(* Logix 5000 AddOnInstructionDefinition export Banner_K50_Select_Touch_PD_v4; software revision 33.03 *)

TYPE Banner_K50Select_Touch_4State_v4 :   // Process Data for Four State Mode.
STRUCT
   PDI_Output_Status : SINT;   // 0 = Inactive, 1 = Active. Related parameters defined in output and touch setting parameter data.
   PDI_State : SINT;   // 0 = State 1, 1 = State 2, 2 = State 3, 3 = State 4. Animation State. Related parameters defined in four state full logic/mulicolor parameter data.
   PDO_Job_Control : SINT;   // 0 = Off, 1 = On. Job input for 4 state full logic mode.
END_STRUCT
END_TYPE

TYPE Banner_K50Select_Touch_Adv_v4 :   // Advanced Process Data information.
STRUCT
   PDI_Output_Status : SINT;   // 0 = Inactive, 1 = Active. Related parameters defined in output and touch settings parameter data.
   Animation_Type : SINT;   // 0 = Off, 1 = Steady, 2 = Flash, 3 = Two Color Flash, 4 = 50/50, 5 = 50/50 Rotate, 6 = Chase, 7 = Intensity Sweep, 8 = Color Sweep, 9 = Sequence, 10 = Wave, 11 = Double Wave.
   Direction : SINT;   // 0 = CCW, 1 = CW.
   Pattern : SINT;   // 0 = Flash, 1 = Strobe, 2 = Three Pulse, 3 = SOS, 4 = Random.
   Speed : SINT;   // 0 = Slow, 1 = Medium, 2 = Fast, 3 = Custom.
   Static_Sequence : INT;   // 0 to 255. Value describing the LED position on the device.
   Sequence_Start_Location : SINT;   // 0 = LED 1, 1 = LED 2, 2 = LED 3, 3 = LED 4, 4 = LED 5, 5 = LED 6, 6 = LED 7, 7 = LED 8.
   Color_1 : SINT;   // 0 = Green, 1 = Red, 2 = Orange, 3 = Amber, 4 = Yellow, 5 = Lime Green, 6 = Spring Green, 7 = Cyan, 8 = Sky Blue, 9 = Blue, 10 = Violet, 11 = Magenta, 12 = Rose, 13 = White, 14 = Custom 1, 15 = Custom 2.
   Color_1_Intensity : SINT;   // 0 = High, 1 = Medium, 2 = Low, 3 = Off, 4 = Custom.
   Color_2 : SINT;   // 0 = Green, 1 = Red, 2 = Orange, 3 = Amber, 4 = Yellow, 5 = Lime Green, 6 = Spring Green, 7 = Cyan, 8 = Sky Blue, 9 = Blue, 10 = Violet, 11 = Magenta, 12 = Rose, 13 = White, 14 = Custom 1, 15 = Custom 2.
   Color_2_Intensity : SINT;   // 0 = High, 1 = Medium, 2 = Low, 3 = Off, 4 = Custom.
END_STRUCT
END_TYPE

TYPE Banner_K50Select_Touch_LEDControl_v4 :   // LED Control Process Data for a K50 Select.
STRUCT
   PDI_Output_Status : SINT;   // 0 = Inactive, 1 = Active. Related parameters defined in output and touch settings parameter data.
   LED_1_Color : SINT;   // 0 = Green, 1 = Red, 2 = Orange, 3 = Amber, 4 = Yellow, 5 = Lime Green, 6 = Spring Green, 7 = Cyan, 8 = Sky Blue, 9 = Blue, 10 = Violet, 11 = Magenta, 12 = Rose, 13 = White, 14 = Custom 1, 15 = Custom 2.
   LED_1_Intensity : SINT;   // 0 to 10 (0 to 100%).
   LED_2_Color : SINT;   // 0 = Green, 1 = Red, 2 = Orange, 3 = Amber, 4 = Yellow, 5 = Lime Green, 6 = Spring Green, 7 = Cyan, 8 = Sky Blue, 9 = Blue, 10 = Violet, 11 = Magenta, 12 = Rose, 13 = White, 14 = Custom 1, 15 = Custom 2.
   LED_2_Intensity : SINT;   // 0 to 10 (0 to 100%).
   LED_3_Color : SINT;   // 0 = Green, 1 = Red, 2 = Orange, 3 = Amber, 4 = Yellow, 5 = Lime Green, 6 = Spring Green, 7 = Cyan, 8 = Sky Blue, 9 = Blue, 10 = Violet, 11 = Magenta, 12 = Rose, 13 = White, 14 = Custom 1, 15 = Custom 2.
   LED_3_Intensity : SINT;   // 0 to 10 (0 to 100%).
   LED_4_Color : SINT;   // 0 = Green, 1 = Red, 2 = Orange, 3 = Amber, 4 = Yellow, 5 = Lime Green, 6 = Spring Green, 7 = Cyan, 8 = Sky Blue, 9 = Blue, 10 = Violet, 11 = Magenta, 12 = Rose, 13 = White, 14 = Custom 1, 15 = Custom 2.
   LED_4_Intensity : SINT;   // 0 to 10 (0 to 100%).
   LED_5_Color : SINT;   // 0 = Green, 1 = Red, 2 = Orange, 3 = Amber, 4 = Yellow, 5 = Lime Green, 6 = Spring Green, 7 = Cyan, 8 = Sky Blue, 9 = Blue, 10 = Violet, 11 = Magenta, 12 = Rose, 13 = White, 14 = Custom 1, 15 = Custom 2.
   LED_5_Intensity : SINT;   // 0 to 10 (0 to 100%).
   LED_6_Color : SINT;   // 0 = Green, 1 = Red, 2 = Orange, 3 = Amber, 4 = Yellow, 5 = Lime Green, 6 = Spring Green, 7 = Cyan, 8 = Sky Blue, 9 = Blue, 10 = Violet, 11 = Magenta, 12 = Rose, 13 = White, 14 = Custom 1, 15 = Custom 2.
   LED_6_Intensity : SINT;   // 0 to 10 (0 to 100%).
   LED_7_Color : SINT;   // 0 = Green, 1 = Red, 2 = Orange, 3 = Amber, 4 = Yellow, 5 = Lime Green, 6 = Spring Green, 7 = Cyan, 8 = Sky Blue, 9 = Blue, 10 = Violet, 11 = Magenta, 12 = Rose, 13 = White, 14 = Custom 1, 15 = Custom 2.
   LED_7_Intensity : SINT;   // 0 to 10 (0 to 100%).
   LED_8_Color : SINT;   // 0 = Green, 1 = Red, 2 = Orange, 3 = Amber, 4 = Yellow, 5 = Lime Green, 6 = Spring Green, 7 = Cyan, 8 = Sky Blue, 9 = Blue, 10 = Violet, 11 = Magenta, 12 = Rose, 13 = White, 14 = Custom 1, 15 = Custom 2.
   LED_8_Intensity : SINT;   // 0 to 10 (0 to 100%).
   Vibration_Feedback : SINT;   // 0 = Off, 1 = On, 2 = Pattern.
   Vibration_Pattern : SINT;   // 0 = Off, 1 = On, 2 = 3 Pulses, 3 = SOS, 4 = Random.
   Vibration_Speed : SINT;   // 0 = Slow, 1 = Medium, 2 = Fast, 3 = Custom.
END_STRUCT
END_TYPE

TYPE Banner_K50Select_Touch_MC_v4 :   // Process Data for Multicolor
STRUCT
   PDI_Output_State : SINT;   // 0 = Inactive, 1 = Active. Related parameters defined in output and touch setting parameter data.
   PDI_State : SINT;   // 0 = State 1, 1 = State 2, 2 = State 3, 3 = State 4. Animation State. Related parameters defined in four state full logic/mulicolor parameter data.
   PDO_State : SINT;   // 0 = State 1, 1 = State 2, 2 = State 3, 3 = State 4. Animation State. Related parameters defined in four state full logic/mulicolor parameter data.
END_STRUCT
END_TYPE

TYPE Banner_K50Select_Touch_PDIO_v4 :   // UDT that records the converted prcoess data.
STRUCT
   PD_MultiColor : Banner_K50Select_Touch_MC_v4;   // Only active when Operation Mode set to 0. State tells the light which of the four states it should be in. 0 = State 1, 1 = State 2, 2 = State 3, 3 = State 4.
   PD_4State : Banner_K50Select_Touch_4State_v4;   // Only active when Operation Mode set to 1. Job Input tells the light how it should behave. 0 - Off, 1 = ON
   PD_Advanced : Banner_K50Select_Touch_Adv_v4;   // Only active when Operation Mode set to 2.
   PD_LED : Banner_K50Select_Touch_LEDControl_v4;   // Only active when Operation Mode set to 3.
   PDO_DT : SINT[8];
   PDI_DT : SINT[2];
END_STRUCT
END_TYPE

ADD_ON_INSTRUCTION Banner_K50_Select_Touch_PD_v4   (* revision 4.0, vendor Banner Engineering *)
// Takes the raw SINT information and converts that data into actual information.
VAR_IN_OUT
   PD : Banner_K50Select_Touch_PDIO_v4; {required}
END_VAR
VAR_INPUT
   Operation_Mode : SINT; {required}   // Linked from Parameters AOI or entered manually.
   Byte_Swap : BOOL; {required}
END_VAR
VAR
   PDO_Temp : SINT[8]; {access None}
   PDI_Temp : SINT[2]; {access None}
END_VAR

ROUTINE Logic   (* ladder *)
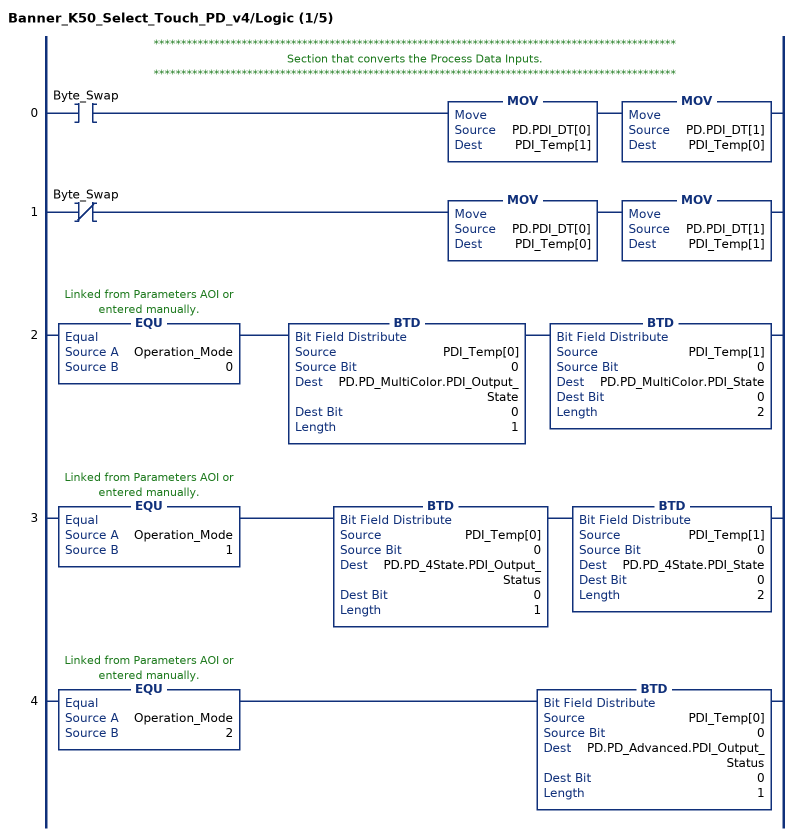
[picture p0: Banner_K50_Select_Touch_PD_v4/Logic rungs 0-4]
   // ***********************************************************************************************
   // Section that converts the Process Data Inputs.
   // ***********************************************************************************************
   0: XIC(Byte_Swap)MOV(PD.PDI_DT[0],PDI_Temp[1])MOV(PD.PDI_DT[1],PDI_Temp[0]);
   1: XIO(Byte_Swap)MOV(PD.PDI_DT[0],PDI_Temp[0])MOV(PD.PDI_DT[1],PDI_Temp[1]);
   2: EQU(Operation_Mode,0)BTD(PDI_Temp[0],0,PD.PD_MultiColor.PDI_Output_State,0,1)BTD(PDI_Temp[1],0,PD.PD_MultiColor.PDI_State,0,2);
   3: EQU(Operation_Mode,1)BTD(PDI_Temp[0],0,PD.PD_4State.PDI_Output_Status,0,1)BTD(PDI_Temp[1],0,PD.PD_4State.PDI_State,0,2);
   4: EQU(Operation_Mode,2)BTD(PDI_Temp[0],0,PD.PD_Advanced.PDI_Output_Status,0,1);
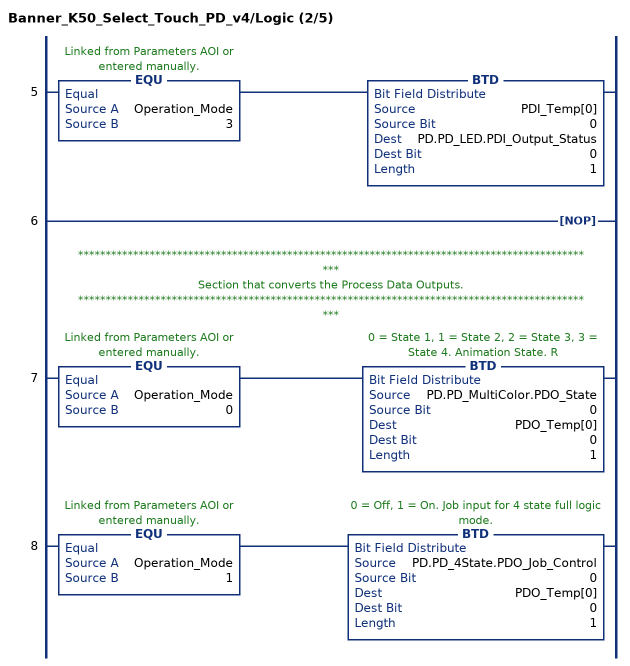
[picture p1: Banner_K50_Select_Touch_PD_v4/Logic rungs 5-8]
   5: EQU(Operation_Mode,3)BTD(PDI_Temp[0],0,PD.PD_LED.PDI_Output_Status,0,1);
   6: NOP();
   // ***********************************************************************************************
   // Section that converts the Process Data Outputs.
   // ***********************************************************************************************
   7: EQU(Operation_Mode,0)BTD(PD.PD_MultiColor.PDO_State,0,PDO_Temp[0],0,1);
   8: EQU(Operation_Mode,1)BTD(PD.PD_4State.PDO_Job_Control,0,PDO_Temp[0],0,1);
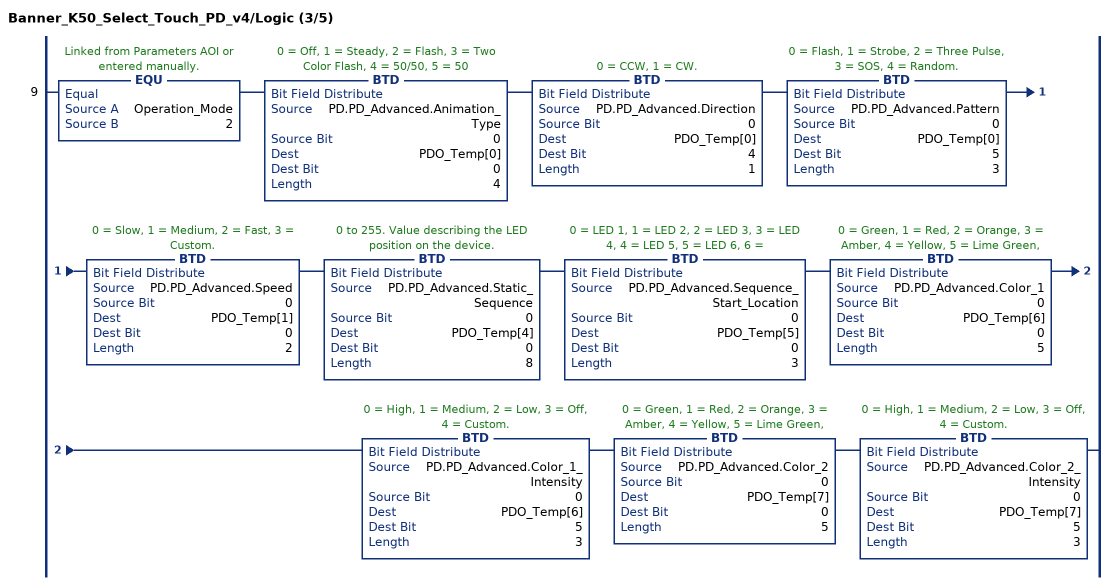
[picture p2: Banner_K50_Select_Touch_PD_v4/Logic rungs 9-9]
   9: EQU(Operation_Mode,2)BTD(PD.PD_Advanced.Animation_Type,0,PDO_Temp[0],0,4)BTD(PD.PD_Advanced.Direction,0,PDO_Temp[0],4,1)BTD(PD.PD_Advanced.Pattern,0,PDO_Temp[0],5,3)BTD(PD.PD_Advanced.Speed,0,PDO_Temp[1],0,2)BTD(PD.PD_Advanced.Static_Sequence,0,PDO_Temp[4],0,8)BTD(PD.PD_Advanced.Sequence_Start_Location,0,PDO_Temp[5],0,3)BTD(PD.PD_Advanced.Color_1,0,PDO_Temp[6],0,5)BTD(PD.PD_Advanced.Color_1_Intensity,0,PDO_Temp[6],5,3)BTD(PD.PD_Advanced.Color_2,0,PDO_Temp[7],0,5)BTD(PD.PD_Advanced.Color_2_Intensity,0,PDO_Temp[7],5,3);
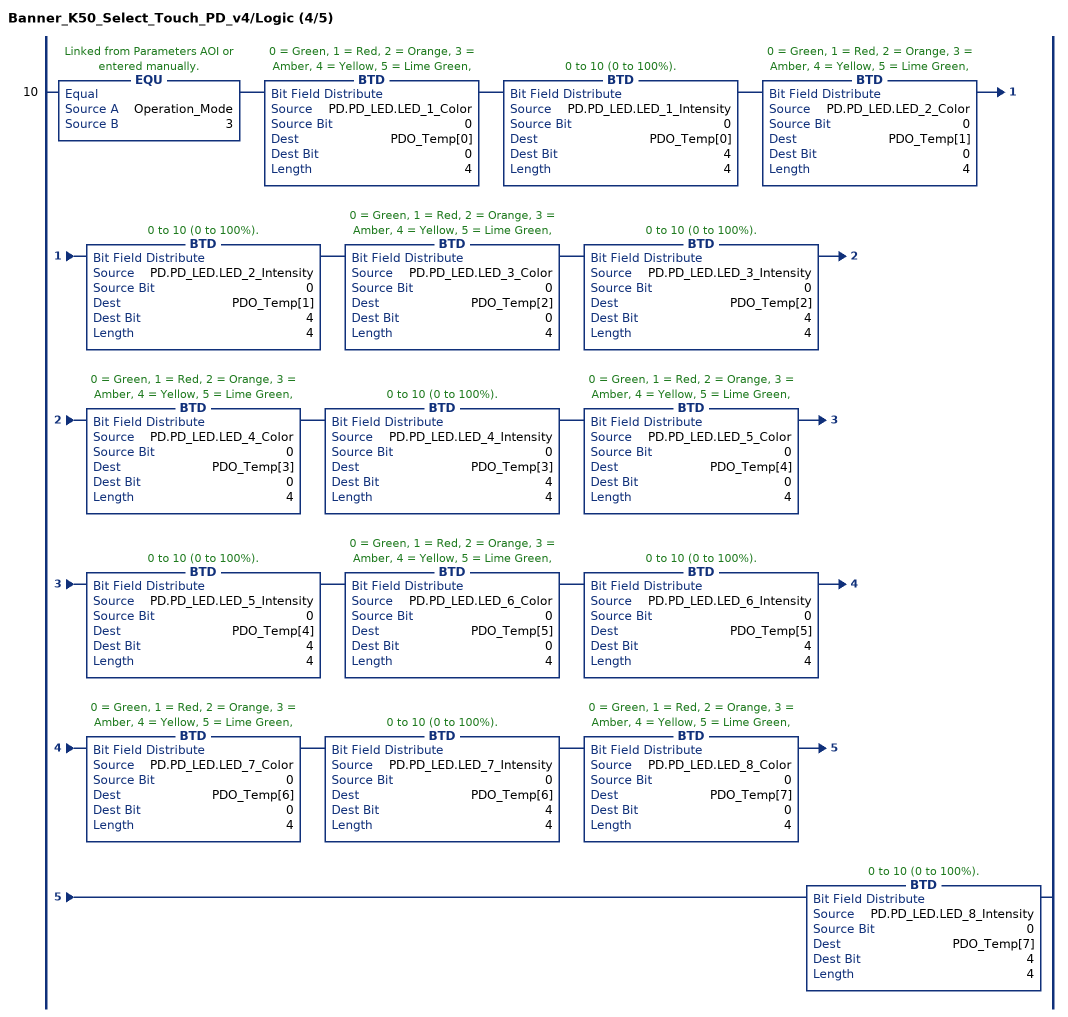
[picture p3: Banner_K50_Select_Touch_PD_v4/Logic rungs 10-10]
   10: EQU(Operation_Mode,3)BTD(PD.PD_LED.LED_1_Color,0,PDO_Temp[0],0,4)BTD(PD.PD_LED.LED_1_Intensity,0,PDO_Temp[0],4,4)BTD(PD.PD_LED.LED_2_Color,0,PDO_Temp[1],0,4)BTD(PD.PD_LED.LED_2_Intensity,0,PDO_Temp[1],4,4)BTD(PD.PD_LED.LED_3_Color,0,PDO_Temp[2],0,4)BTD(PD.PD_LED.LED_3_Intensity,0,PDO_Temp[2],4,4)BTD(PD.PD_LED.LED_4_Color,0,PDO_Temp[3],0,4)BTD(PD.PD_LED.LED_4_Intensity,0,PDO_Temp[3],4,4)BTD(PD.PD_LED.LED_5_Color,0,PDO_Temp[4],0,4)BTD(PD.PD_LED.LED_5_Intensity,0,PDO_Temp[4],4,4)BTD(PD.PD_LED.LED_6_Color,0,PDO_Temp[5],0,4)BTD(PD.PD_LED.LED_6_Intensity,0,PDO_Temp[5],4,4)BTD(PD.PD_LED.LED_7_Color,0,PDO_Temp[6],0,4)BTD(PD.PD_LED.LED_7_Intensity,0,PDO_Temp[6],4,4)BTD(PD.PD_LED.LED_8_Color,0,PDO_Temp[7],0,4)BTD(PD.PD_LED.LED_8_Intensity,0,PDO_Temp[7],4,4);
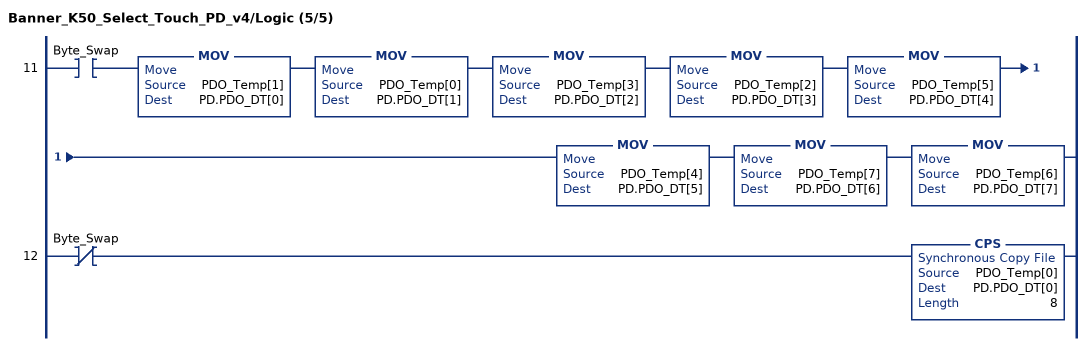
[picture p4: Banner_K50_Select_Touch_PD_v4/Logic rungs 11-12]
   11: XIC(Byte_Swap)MOV(PDO_Temp[1],PD.PDO_DT[0])MOV(PDO_Temp[0],PD.PDO_DT[1])MOV(PDO_Temp[3],PD.PDO_DT[2])MOV(PDO_Temp[2],PD.PDO_DT[3])MOV(PDO_Temp[5],PD.PDO_DT[4])MOV(PDO_Temp[4],PD.PDO_DT[5])MOV(PDO_Temp[7],PD.PDO_DT[6])MOV(PDO_Temp[6],PD.PDO_DT[7]);
   12: XIO(Byte_Swap)CPS(PDO_Temp[0],PD.PDO_DT[0],8);
END_ROUTINE
END_ADD_ON_INSTRUCTION
